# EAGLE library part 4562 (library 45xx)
128-bit static SHIFT REGISTER
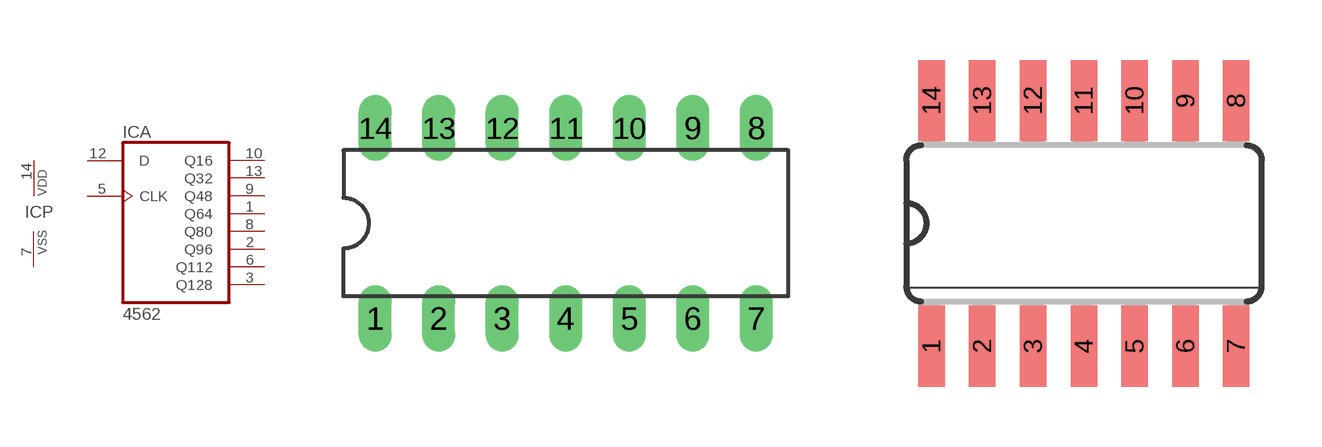
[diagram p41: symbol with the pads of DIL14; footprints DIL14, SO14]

Designator prefix IC; gates A=4562 P=PWRN

## 4562N  [DIL14]
1  A:Q64  out
2  A:Q96  out
3  A:Q128  out
5  A:CLK  in
6  A:Q112  out
7  P:VSS  pwr
8  A:Q80  out
9  A:Q48  out
10  A:Q16  out
12  A:D  in
13  A:Q32  out
14  P:VDD  pwr

## 4562D  [SO14]
Pads as for DIL14

## Footprint DIL14 (pad centres in mm)
Dual In Line Package
drill 0.813 long: 1 -7.62,-3.81; 2 -5.08,-3.81; 3 -2.54,-3.81; 4 0,-3.81; 5 2.54,-3.81; 6 5.08,-3.81; 7 7.62,-3.81; 8 7.62,3.81; 9 5.08,3.81; 10 2.54,3.81; 11 0,3.81; 12 -2.54,3.81; 13 -5.08,3.81; 14 -7.62,3.81

## Footprint SO14 (pad centres in mm)
Small Outline package 150 mil
smd 0.66 x 2.032: 1 -3.81,-3.073; 2 -2.54,-3.073; 3 -1.27,-3.073; 4 0,-3.073; 5 1.27,-3.073; 6 2.54,-3.073; 7 3.81,-3.073; 8 3.81,3.073; 9 2.54,3.073; 10 1.27,3.073; 11 0,3.073; 12 -1.27,3.073; 13 -2.54,3.073; 14 -3.81,3.073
